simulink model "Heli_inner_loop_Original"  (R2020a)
settings: Solver=FixedStepDiscrete  StartTime=0.0  StopTime=10.0  FixedStep=0.01  RelTol=1e-3  EnableMultiTasking=on

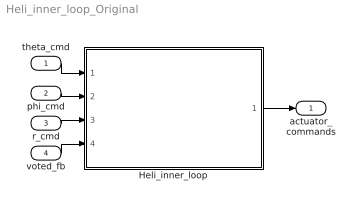
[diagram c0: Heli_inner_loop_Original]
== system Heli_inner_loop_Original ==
  theta_cmd : Inport  OutMin=-30  OutMax=30  OutDataTypeStr=double  PortDimensions=1  SampleTime=0.01
  phi_cmd : Inport  Port=2  OutMin=-30  OutMax=30  OutDataTypeStr=double  PortDimensions=1  SampleTime=0.01
  r_cmd : Inport  Port=3  OutMin=-30  OutMax=30  OutDataTypeStr=double  PortDimensions=1  SampleTime=0.01
  voted_fb : Inport  Port=4  OutMin=-180  OutMax=180  OutDataTypeStr=double  PortDimensions=5  SampleTime=0.01
  Heli_inner_loop : ModelReference  ModelNameDialog=Heli_inner_loop  SimulationMode=Normal  ModelReferenceVersion=1.32
  actuator_commands : Outport  VectorParamsAs1DForOutWhenUnconnected=off
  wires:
  theta_cmd/1 -> Heli_inner_loop/1
  phi_cmd/1 -> Heli_inner_loop/2
  r_cmd/1 -> Heli_inner_loop/3
  voted_fb/1 -> Heli_inner_loop/4
  Heli_inner_loop/1 -> actuator_commands/1
